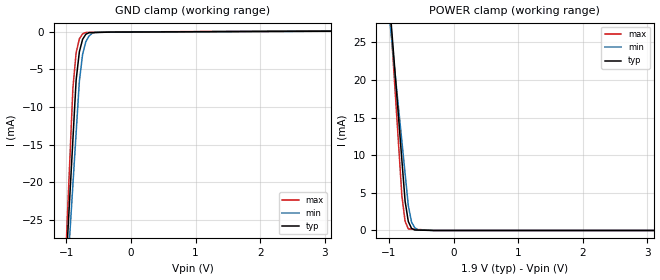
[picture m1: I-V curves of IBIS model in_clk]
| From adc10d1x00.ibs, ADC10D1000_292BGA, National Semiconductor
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[Model] in_clk
Model_type Input
Vinl = 400.000mV
Vinh = 2.00000V
C_comp 1.05pF 1.05pF 1.05pF
| variable typ   min   max
[Voltage Range] 1.90000V 1.80000V 2.00000V
[POWER Clamp Reference] 1.90000V 1.80000V 2.00000V
[GND Clamp Reference] 0.00000V 0.00000V 0.00000V
[Temperature Range]   25   85   -40
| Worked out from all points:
|   GND clamp passes 1 mA (typ) near -0.75 V on its own axis
|   POWER clamp passes 1 mA (typ) near -0.69 V on its own axis
[GND Clamp]
-1.9V     -171.8mA   -157.6mA   -207.7mA
-900mV    -14.3mA    -20.28mA   -7.454mA
-850mV    -6.422mA   -13.42mA   -2.791mA
-800mV    -2.667mA   -6.555mA   -951.9uA
-750mV    -1.012mA   -3.013mA   -278uA
-700mV    -338.5uA   -1.319mA   -99.95uA
-650mV    -130.8uA   -564.6uA   -92.55uA
-600mV    -118.7uA   -203.2uA   -85.15uA
-550mV    -106.5uA   -90.23uA   -77.75uA
3.8V      89.25uA    98.44uA    155.4uA
[POWER Clamp]
-1.9V     130.3mA    106.3mA    151.5mA
-900mV    20.38mA    20.45mA    17.99mA
-800mV    9.389mA    11.86mA    4.646mA
-750mV    3.894mA    7.571mA    1.226mA
-700mV    1.187mA    3.278mA    205.6uA
-650mV    275.1uA    1.111mA    179.9uA
-600mV    61.9uA     352.7uA    154.2uA
-550mV    51.58uA    88.51uA    128.5uA
-300mV    0A         0A         0A
3.8V      0A         0A         0A
